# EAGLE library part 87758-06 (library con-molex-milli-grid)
HEADER
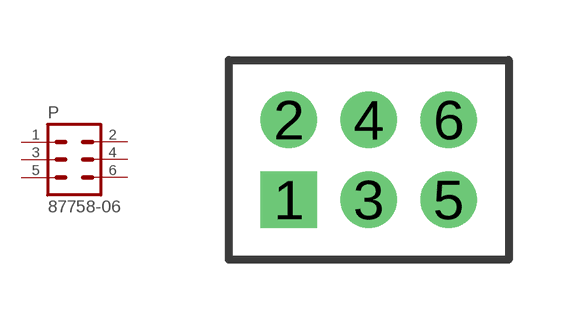
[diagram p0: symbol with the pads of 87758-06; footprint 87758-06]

Designator prefix P

## 87758-06  [87758-06]
1  1  pas
2  2  pas
3  3  pas
4  4  pas
5  5  pas
6  6  pas

## Footprint 87758-06 (pad centres in mm)
HEADER Dual Row, Vertical
drill 0.914 square: 1 -2,-1
drill 0.914: 2 -2,1; 3 0,-1; 4 0,1; 5 2,-1; 6 2,1

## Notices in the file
Copyright (C) 2010, Bob Starr
